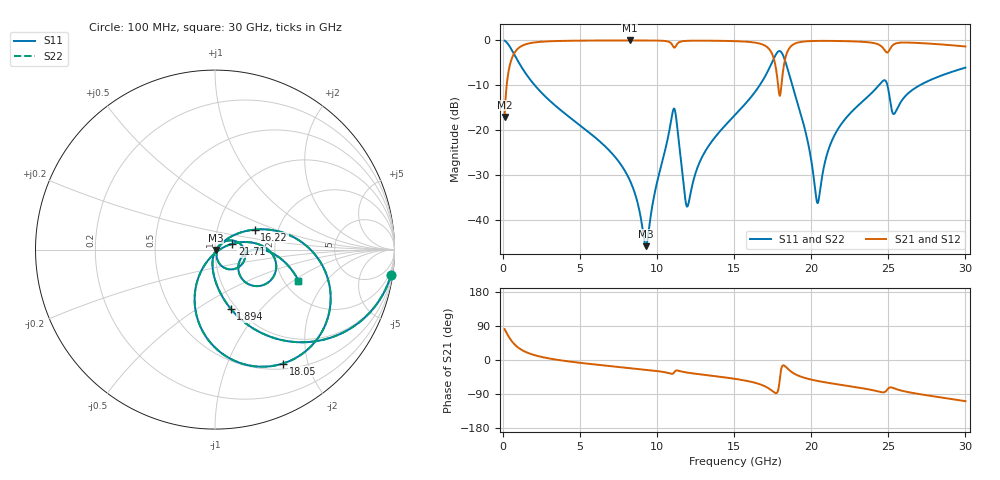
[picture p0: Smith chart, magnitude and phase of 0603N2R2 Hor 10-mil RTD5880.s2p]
# GHz S MA R 50
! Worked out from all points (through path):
!   3201 points, 100 MHz to 30 GHz, reference 50 ohm
!   highest |S21| = -0.04 dB at 8.21 GHz (marker M1); lowest = -17.1 dB at 100 MHz (marker M2)
!   group delay of S21, straight-line fit = 11.3 ps
!   lowest |S11| = -45.8 dB at 9.266 GHz (marker M3), VSWR 1.01, Z = 50.4 - j0.253 ohm
!   |S11| at or under -10 dB: 2.053 GHz to 16.66 GHz (14.6 GHz wide, 156 % of centre); 18.77 GHz to 24.39 GHz (5.618 GHz wide, 26 % of centre); 24.94 GHz to 27.04 GHz (2.104 GHz wide, 8.1 % of centre)
!   |S22| runs from -45.8 to -0.1 dB; largest |S21 - S12| = 0
!   S11 on the Smith chart (normalised r, x): 100 MHz: 1, -14; 1.894 GHz: 0.94, -0.70; 16.22 GHz: 1.52, +0.36; 18.05 GHz: 0.58, -1.61; 21.71 GHz: 1.21, +0.08; 30 GHz: 2.39, -1.09
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0.1  0.9901 -8.3  0.1403 81.6  0.1403 81.6  0.9901 -8.3
0.6325937  0.7434 -43.7  0.6682 46.3  0.6682 46.3  0.7434 -43.7
1.894  0.3412 -75.1  0.9385 14.7  0.9385 14.7  0.3412 -75.1
5.089563  0.1099 -96.5  0.9912 -7.9  0.9912 -7.9  0.1099 -96.5
8.210375  0.02802 -103.0  0.9955 -21.2  0.9955 -21.2  0.02802 -103.0
9.266219  0.005114 -29.3  0.9948 -25.7  0.9948 -25.7  0.005114 -29.3
10.06978  0.02986 44.6  0.9913 -29.6  0.9913 -29.6  0.02986 44.6
11.06022  0.1713 -9.2  0.8426 -34.8  0.8426 -34.8  0.1713 -9.2
11.95722  0.01412 -15.6  0.9864 -33.3  0.9864 -33.3  0.01412 -15.6
13.00372  0.05368 42.3  0.9901 -38.9  0.9901 -38.9  0.05368 42.3
15.05  0.1475 36.0  0.978 -49.7  0.978 -49.7  0.1475 36.0
16.21797  0.2486 26.7  0.9485 -58.7  0.9485 -58.7  0.2486 26.7
17.32988  0.5112 2.2  0.7725 -77.5  0.7725 -77.5  0.5112 2.2
17.75034  0.7148 -26.1  0.4337 -87.1  0.4337 -87.1  0.7148 -26.1
18.04934  0.7392 -59.2  0.3006 -23.9  0.3006 -23.9  0.7392 -59.2
18.60997  0.3939 -104.5  0.8313 -28.1  0.8313 -28.1  0.3939 -104.5
20.03956  0.04164 -116.6  0.9811 -52.1  0.9811 -52.1  0.04164 -116.6
20.44134  0.01572 -41.0  0.9845 -55.5  0.9845 -55.5  0.01572 -41.0
21.71209  0.1015 18.6  0.9821 -64.3  0.9821 -64.3  0.1015 18.6
25.01978  0.2709 -45.7  0.7533 -74.2  0.7533 -74.2  0.2709 -45.7
25.39353  0.1525 -18.5  0.9076 -75.0  0.9076 -75.0  0.1525 -18.5
30  0.496 -20.3  0.853 -108.6  0.853 -108.6  0.496 -20.3
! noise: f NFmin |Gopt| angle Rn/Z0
0.1  0.0004443  0.9476  0.8889  0.001901
3.417  0.004024  0.8095  9.794  0.004369
6.743  0.006966  0.7865  18.89  0.006533
10.06  0.01327  0.83  27.85  0.0155
13.39  0.01536  0.8087  36.77  0.01507
16.7  0.03504  0.8918  45.51  0.06
20.03  0.02761  0.8416  54.29  0.02933
23.35  0.02884  0.8269  62.42  0.02573
26.67  0.03327  0.8305  70.55  0.0277
30  0.03258  0.8104  78.13  0.02174
